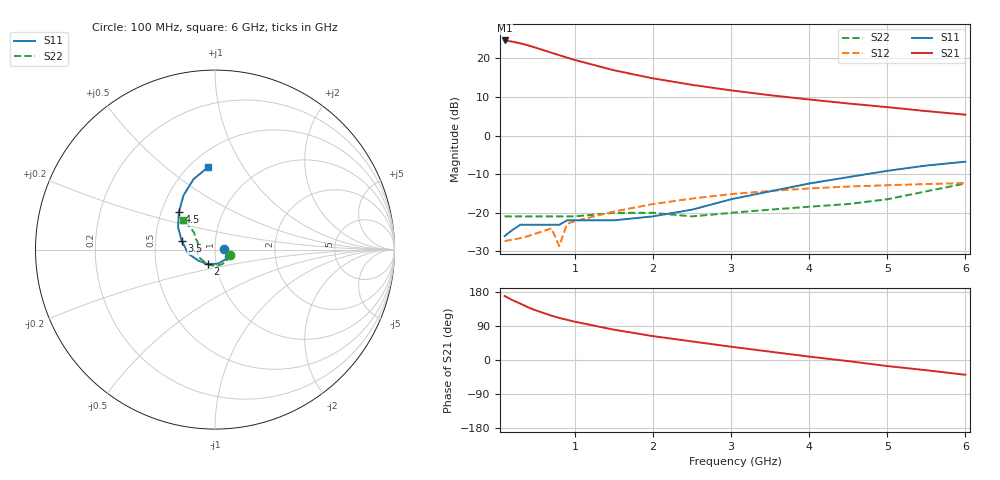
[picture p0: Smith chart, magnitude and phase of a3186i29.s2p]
!  MSA-3186 S AND NOISE PARAMETERS
!  Id = 29 mA  LAST UPDATED 06-27-94
# ghz s ma r 50
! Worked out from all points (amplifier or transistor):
!   20 points, 100 MHz to 6 GHz, reference 50 ohm
!   highest |S21| = 24.7 dB at 100 MHz (marker M1)
!   |S21| within 3 dB of that: start of sweep to 672 MHz
!   unconditionally stable (mu >= 1): start of sweep to end of sweep
!   at 400 MHz: K = 1.04, MAG = 23.5 dB, |S12| = -26.0 dB
!   at 1.5 GHz: K = 1.03, MAG = 17.2 dB, |S12| = -19.7 dB
!   at 6 GHz: K = 1.02, MAG = 7.9 dB, |S12| = -12.3 dB
!   S11 on the Smith chart (normalised r, x): 100 MHz: 1.11, +0.00; 2 GHz: 0.91, -0.15; 3.5 GHz: 0.69, +0.07; 4.5 GHz: 0.62, +0.28; 6 GHz: 0.61, +0.71
0.1  0.05 1.0  17.11 169.0  0.043 7.0  0.09 -19.0
0.2  0.06 2.0  16.52 158.0  0.045 14.0  0.09 -37.0
0.3  0.07 -2.0  15.72 149.0  0.047 20.0  0.09 -52.0
0.4  0.07 -7.0  14.77 139.0  0.05 24.0  0.09 -67.0
0.5  0.07 -12.0  13.77 131.0  0.054 29.0  0.09 -80.0
0.6  0.07 -21.0  12.79 124.0  0.058 32.0  0.09 -92.0
0.7  0.07 -27.0  11.86 117.0  0.063 34.0  0.09 -102.0
0.8  0.07 -33.0  11.03 111.0  0.037 36.0  0.09 -111.0
0.9  0.08 -39.0  10.25 106.0  0.072 38.0  0.09 -119.0
1  0.08 -44.0  9.55 101.0  0.078 39.0  0.09 -127.0
1.5  0.08 -79.0  7.03 80.0  0.104 39.0  0.1 -155.0
2  0.09 -116.0  5.52 63.0  0.13 36.0  0.1 -171.0
2.5  0.11 -145.0  4.55 49.0  0.153 31.0  0.09 176.0
3  0.15 -171.0  3.86 35.0  0.175 25.0  0.1 162.0
3.5  0.19 166.0  3.34 22.0  0.192 19.0  0.11 154.0
4  0.24 149.0  2.94 9.0  0.207 13.0  0.12 152.0
4.5  0.29 134.0  2.61 -3.0  0.219 7.0  0.13 148.0
5  0.35 120.0  2.34 -16.0  0.228 1.0  0.15 141.0
5.5  0.41 107.0  2.08 -27.0  0.236 -5.0  0.19 138.0
6  0.46 95.0  1.87 -39.0  0.243 -10.0  0.24 137.0
